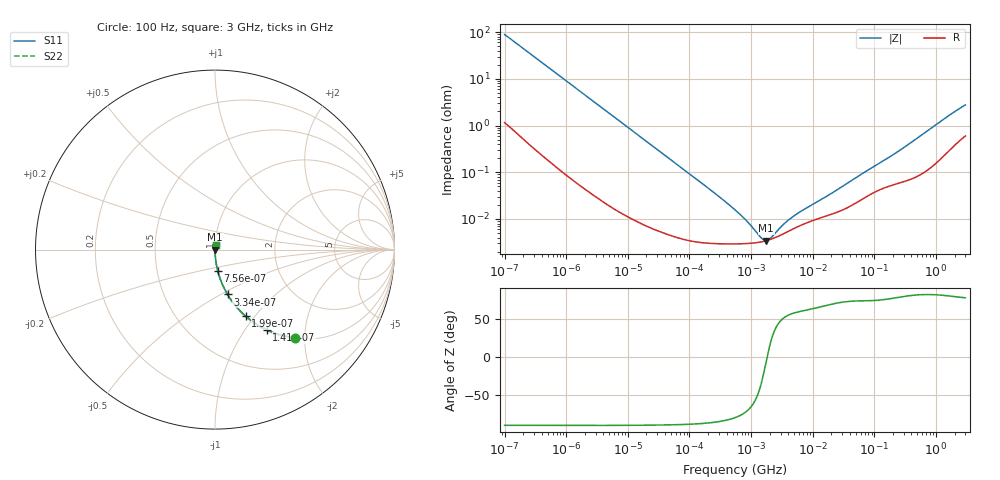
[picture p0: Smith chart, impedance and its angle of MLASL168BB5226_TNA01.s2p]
! MLASL168BB5226_TNA01  S-PARAMETER MODEL  ( Standard Model )
! Model Generated by TAIYO YUDEN Corporation (http://www.ty-top.com)
! Version 2.0
! TAIYO YUDEN Control No. 230906
! Copyright(c) 2016 TAIYO YUDEN CO.,LTD. All Rights Reserved.
! Product Description (link to TY-COMPAS)
! https://ds.yuden.co.jp/TYCOMPAS/or/detail?pn=MLASL168BB5226MTNA01&u=M
! Products Name : Multilayer Ceramic Capacitors
! Characteristics :
!  Capacitance : 22 [uF] , Rated Voltage : 10 [V] , TCC : X5R
!  Case Size : 1.6 x 0.8 / 0.063 x 0.031 [mm/inch] , Thickness : 0.8 / 0.031 [mm/inch]
!  (Conditions: Temperature = 25 [degC] , DC Bias Voltage = 0 [V])
! External Node Assignments :
!  1  o---| |---o  2
! GND o---------o GND
! Frequency Range : 100Hz  -  3GHz  [ 401 STEP ]
# MHZ S RI R 50
! Freq[MHz].  S11 Real  S11 Imag  S21 Real  S21 Imag  S12 Real  S12 Imag  S22 Real  S22 Imag
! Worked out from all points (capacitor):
!   401 points, 100 Hz to 3 GHz, reference 50 ohm
!   read as one part in series: C = 17.8 uF near 109 Hz
!   lowest |Z| = 3.45 mohm at 1.751 MHz (marker M1)
!   series resonance near 1.82 MHz, so ESL is about 430 pH
!   S11 on the Smith chart (normalised r, x): 100 Hz: 1.02, -1.78; 141 Hz: 1.02, -1.27; 199 Hz: 1.01, -0.90; 334 Hz: 1.01, -0.54; 756 Hz: 1.00, -0.24; 3 GHz: 1.01, +0.05
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0.0001  0.4429 -0.4903  0.5571 0.4903  0.5571 0.4903  0.4429 -0.4903
0.000141  0.2885 -0.4469  0.7115 0.4469  0.7115 0.4469  0.2885 -0.4469
0.000199  0.1712 -0.371  0.8288 0.371  0.8288 0.371  0.1712 -0.371
0.000334  0.0699 -0.2498  0.9301 0.2498  0.9301 0.2498  0.0699 -0.2498
0.000513  0.0315 -0.1697  0.9685 0.1697  0.9685 0.1697  0.0315 -0.1697
0.000756  0.0152 -0.1175  0.9848 0.1175  0.9848 0.1175  0.0152 -0.1175
0.001788  0.00305 -0.0506  0.9969 0.0506  0.9969 0.0506  0.00305 -0.0506
0.005476  0.000454 -0.0167  0.9995 0.0167  0.9995 0.0167  0.000454 -0.0167
0.031977  6.29e-05 -0.00288  0.9999 0.00288  0.9999 0.00288  6.29e-05 -0.00288
0.221826  3.02e-05 -0.000413  1 0.000413  1 0.000413  3.02e-05 -0.000413
0.547723  2.93e-05 -0.000155  1 0.000155  1 0.000155  2.93e-05 -0.000155
0.740304  2.96e-05 -0.000105  1 0.000105  1 0.000105  2.96e-05 -0.000105
0.842342  2.98e-05 -8.67e-05  1 8.67e-05  1 8.67e-05  2.98e-05 -8.67e-05
1.75092  3.42e-05 -3.84e-06  1 3.84e-06  1 3.84e-06  3.42e-05 -3.84e-06
4.141163  5.56e-05 8.04e-05  0.9999 -8.04e-05  0.9999 -8.04e-05  5.56e-05 8.04e-05
9.794414  9.18e-05 0.000181  0.9999 -0.000181  0.9999 -0.000181  9.18e-05 0.000181
20.35898  0.000127 0.000333  0.9999 -0.000333  0.9999 -0.000333  0.000127 0.000333
65.08213  0.000271 0.000914  0.9997 -0.000914  0.9997 -0.000914  0.000271 0.000914
175.1444  0.000509 0.00205  0.9995 -0.00205  0.9995 -0.00205  0.000509 0.00205
348.7234  0.000685 0.0038  0.9993 -0.0038  0.9993 -0.0038  0.000685 0.0038
1573.002  0.00299 0.0156  0.997 -0.0156  0.997 -0.0156  0.00299 0.0156
3000  0.00666 0.0268  0.9933 -0.0268  0.9933 -0.0268  0.00666 0.0268
